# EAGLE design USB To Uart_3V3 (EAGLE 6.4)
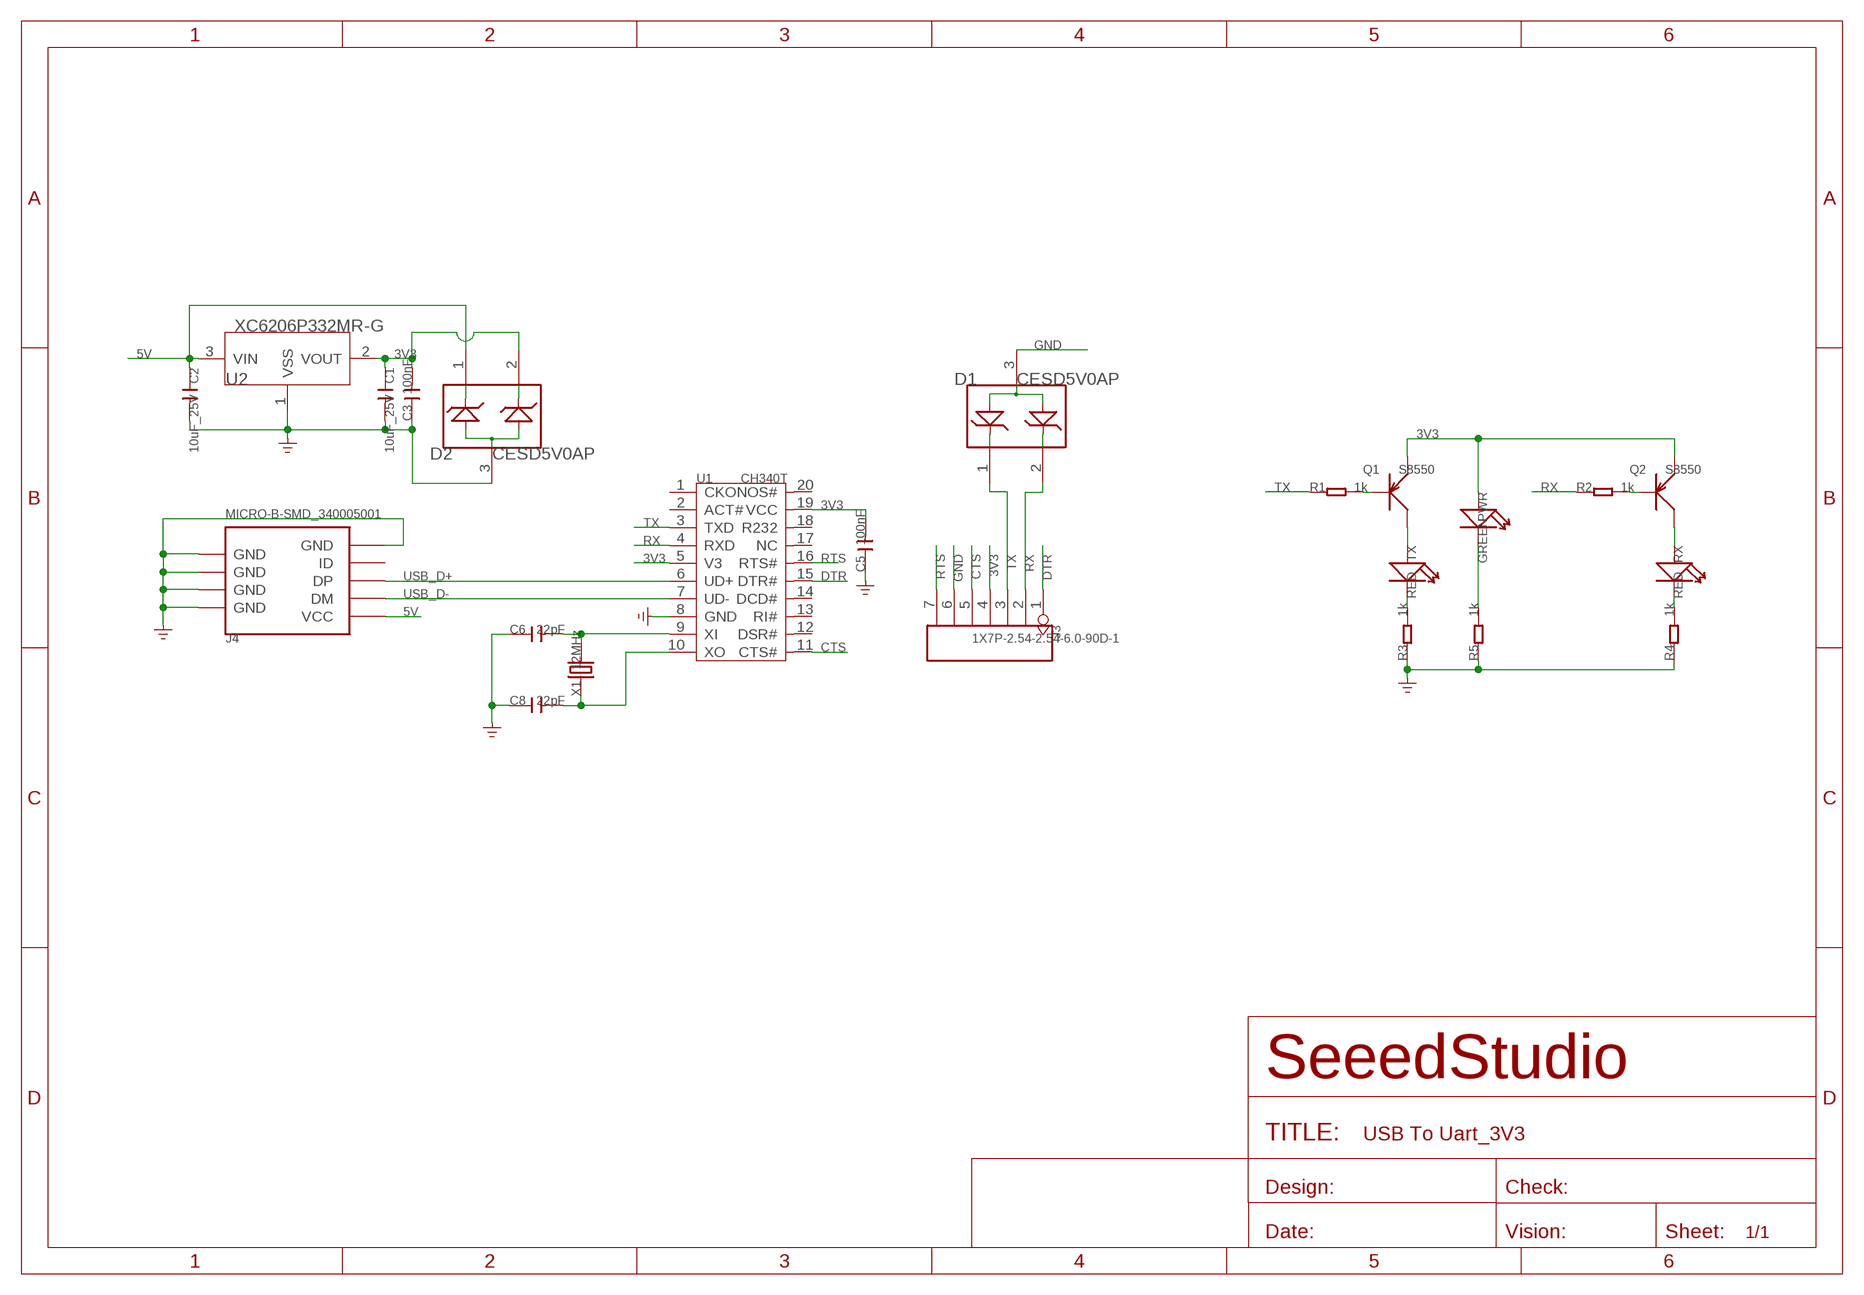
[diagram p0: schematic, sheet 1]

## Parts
C1  10uF_25V  C-0805  [C0805]
C2  10uF_25V  C-0805  [C0805]
C3  100nF  C-0402  [C0402]
C5  100nF  C-0402  [C0402]
C6  22pF  C-0402  [C0402]
C8  22pF  C-0402  [C0402]
D1  CESD5V0AP  D-ESD-3P  [SOT23]
D2  CESD5V0AP  D-ESD-3P  [SOT23]
J3  1X7P-2.54-2.54-6.0-90D-1  HEADER-7P  [7P-2.54-65/35MIL]
J4  MICRO-B-SMD_340005001  USB-MINIUSB-5P-MICRO  [MICRO-USB]
PWR  GREEN  LED'0603'  [LED-0603]
Q1  S8550  TRANSISTOR-PNP-SOT23  [SOT23]
Q2  S8550  TRANSISTOR-PNP-SOT23  [SOT23]
R1  1k  R-0402  [R0402]
R2  1k  R-0402  [R0402]
R3  1k  R-0402  [R0402]
R4  1k  R-0402  [R0402]
R5  1k  R-0402  [R0402]
RX  RED  LED'0603'  [LED-0603]
TX  RED  LED'0603'  [LED-0603]
U1  CH340T  [SSOP20]
U2  XC6206P332MR-G  XC6206MR  [SOT23]
X1  12MHz  CRYSTAL'HC49UP'  [HC49UP]

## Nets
3V3: C1.1 C3.2 C5.2 D2.2 J3.4 PWR.+ Q1.2(E) Q2.2(E) U1.5(V3) U1.19(VCC) U2.2(VOUT)
5V: C2.1 D2.1 J4.1(VCC) U2.3(VIN)
CTS: J3.5 U1.11(CTS#)
DTR: J3.1 U1.15(DTR#)
GND: C1.2 C2.2 C3.1 C5.1 C6.1 C8.1 D1.3 D2.3 J3.6 J4.5(GND) J4.S1(GND) J4.S2(GND) J4.S3(GND) J4.S4(GND) J4.S5(GND) J4.S6(GND) R3.1 R4.1 R5.1 U1.8(GND) U2.1(VSS)
N$1: Q1.3(C) TX.+
N$2: Q2.3(C) RX.+
N$4: C6.2 U1.9(XI) X1.2
N$5: C8.2 U1.10(XO) X1.1
N$6: R3.2 TX.-
N$7: Q1.1(B) R1.2
N$8: Q2.1(B) R2.2
N$10: R4.2 RX.-
N$12: PWR.- R5.2
RTS: J3.7 U1.16(RTS#)
RX: D1.2 J3.2 R2.1 U1.4(RXD)
TX: D1.1 J3.3 R1.1 U1.3(TXD)
USB_D+: J4.3(DP) U1.6(UD+)
USB_D-: J4.2(DM) U1.7(UD-)
Unconnected: J4.4(ID) U1.1(CKO) U1.2(ACT#) U1.12(DSR#) U1.13(RI#) U1.14(DCD#) U1.17(NC) U1.18(R232) U1.20(NOS#)

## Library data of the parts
C1-C3 C5 C6 C8 = Discrete:C*: Ceramic Capacitors
D1 D2 = Discrete:D-ESD-3P
J3 = Connector :HEADER-7P
J4 = Connector :USB-MINIUSB-5P
PWR RX TX = Discrete:LED*
Q1 Q2 = Discrete:TRANSISTOR-PNP*: PNP audion
R1-R5 = Discrete:R*
U1 = template:CH340T
U2 = IC:XC6206: LOW ESR Cap.Compatible Positive Voltage Regulators
X1 = Discrete:CRYSTAL*: CRYSTAL

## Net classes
0 default: width 0.152 mm, drill 0.305 mm, clearance 0.152 mm

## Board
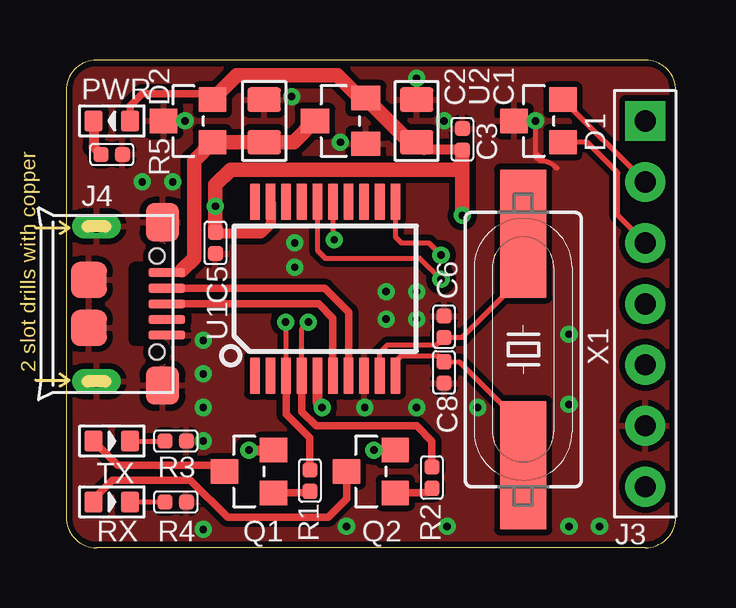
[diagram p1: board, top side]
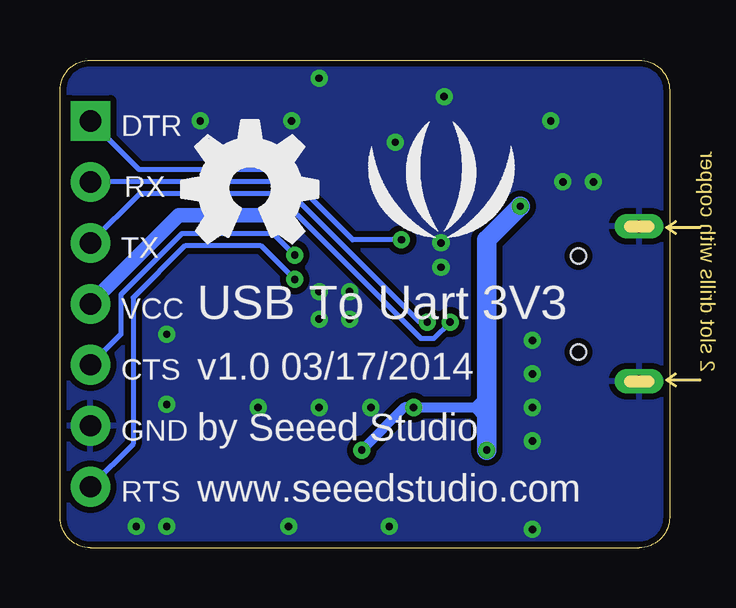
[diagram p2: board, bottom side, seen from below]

Size 25.4 x 20.32 mm. Coordinates in mm from the lower left corner, seen from the top.
Outline: 0,19.05 0,1.27 arc90 1.27,0 24.13,0 arc90 25.4,1.27 25.4,19.05 arc90 24.13,20.32 1.27,20.32 arc90 0,19.05
Copper layers (1*16): Top 0.035mm / dielectric 1.5mm / Bottom 0.035mm
Design rules "default *": minimum track width 8mil, minimum drill 12mil, track to track 8mil, track to pad 8mil, pad to pad 8mil, via to via 8mil, smd to smd 0mil, copper to edge 8mil, drill to drill 8mil, minimum pad ring 10mil, minimum via ring 8mil, stop-mask expansion 4mil, vias tented up to drill 25mil, thermal gap 10mil

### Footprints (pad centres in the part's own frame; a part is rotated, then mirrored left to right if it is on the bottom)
C0805 = smd 1.016 x 1.397: 1 -0.889,0; 2 0.889,0
C0402 = smd 0.635 x 0.635: 1 -0.445,0; 2 0.445,0
SOT23 = smd 1.016 x 1.143: 1 -0.889,-1.016; 2 0.889,-1.016; 3 0,1.016
7P-2.54-65/35MIL = drill 0.889 pad 1.651 square: 1 0,7.62 | drill 0.889 pad 1.651: 2 0,5.08; 3 0,2.54; 4 0,0; 5 0,-2.54; 6 0,-5.08; 7 0,-7.62
MICRO-USB = smd 0.381 x 1.524: 1 -1.3,-0.25; 2 -0.65,-0.25; 3 0,-0.25; 4 0.65,-0.25; 5 1.3,-0.25 | smd 1.6 x 1.397: S1 -3.4,-0.427; S6 3.4,-0.427 | drill 0.508 pad 1.016 long: S2 -3.226,-3.175; S5 3.226,-3.175 | smd 1.5 x 1.5: S3 -1,-3.5; S4 1,-3.5 | hole 0.635: -2,-0.65; 2,-0.65
LED-0603 = smd 0.762 x 0.889: + -0.762,0; - 0.762,0
R0402 = smd 0.635 x 0.635: 1 -0.445,0; 2 0.445,0
SSOP20 = smd 0.4 x 1.5: 1 -2.925,-3.625; 2 -2.275,-3.625; 3 -1.625,-3.625; 4 -0.975,-3.625; 5 -0.325,-3.625; 6 0.325,-3.625; 7 0.975,-3.625; 8 1.625,-3.625; 9 2.275,-3.625; 10 2.925,-3.625; 11 2.925,3.625; 12 2.275,3.625; 13 1.625,3.625; 14 0.975,3.625; 15 0.325,3.625; 16 -0.325,3.625; 17 -0.975,3.625; 18 -1.625,3.625; 19 -2.275,3.625; 20 -2.925,3.625
SOT23' = smd 1.016 x 1.2: 1 -0.95,-1.06; 2 0.95,-1.06; 3 0,1.06
HC49UP = smd 5.334 x 1.93: 1 -4.826,0; 2 4.826,0

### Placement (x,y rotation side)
C1  14.61,17.78 90 top
C2  8.26,17.78 90 top
C3  16.51,17.02 270 top
C5  6.22,12.7 90 top
C6  15.75,9.21 270 top
C8  15.75,7.3 90 top
D1  19.68,17.78 90 top
D2  5.08,17.78 90 top
J3  24.13,10.16 0 top
J4  4.45,10.16 270 top
PWR  1.91,17.78 180 top
Q1  7.62,3.17 90 top
Q2  12.7,3.17 90 top
R1  10.16,2.79 270 top
R2  15.24,2.92 270 top
R3  4.57,4.45 180 top
R4  4.57,1.91 180 top
R5  1.91,16.38 180 top
RX  1.91,1.91 0 top
TX  1.91,4.45 0 top
U1  10.79,10.79 0 top
U2  XC6206P332MR-G  [SOT23']  11.43,17.78 90 top
U$8  [LOGO_SILK]  9.53,14.61 0 bottom
U$9  [OSHW_FILLX200_NOTEXT]  20.32,12.7 0 bottom
X1  19.05,8.26 90 top

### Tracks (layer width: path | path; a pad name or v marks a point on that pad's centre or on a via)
3V3  (via drill 0.3, 0.3 pad 0.64)
  Top 0.305: D2.2 5.84,18.92 3.17,18.92 2.67,18.41 PWR.+
  Top 0.406: Q2.2 v12.83,4.06 | v7.62,4.06 Q1.2 | U1.5 10.47,6.04 v10.67,5.84 | U1.19 8.52,13.47 8.13,13.08 6.29,13.08 C5.2 | C3.2 14.92,16.57 C1.1
  Top 0.61: C1.1 14.33,16.89 U2.2 12.26,18.73 11.3,19.68 7.11,19.68 D2.2 | C3.2 16.51,16 | 16.51,16 16.26,15.75 6.86,15.75 6.22,15.11 v6.22,14.22 C5.2 | 16.51,16 v16.51,13.84
  Bottom 0.406: 8.13,5.84 v10.67,5.84 11.05,5.84 v12.83,4.06 | 8.13,5.84 7.62,6.35 | 8.13,5.84 7.75,5.46
  Bottom 0.61: v16.51,13.84 20.45,13.84 J3.4
  Bottom 0.813: v7.62,4.06 7.62,6.35 7.62,12.83 v6.22,14.22
5V
  Top 0.203: J4.1 4.73,11.46 4.83,11.56
  Top 0.61: 4.83,11.56 5.33,12.06 5.33,16.13 D2.1 C2.1 9.48,16.89 U2.3
CTS  (via drill 0.3)
  Top 0.203: U1.11 13.72,12.95 13.97,12.7 15.11,12.7 v15.62,12.19
  Bottom 0.203: v15.62,12.19 16.51,13.08 20.32,13.08 22.86,10.54 22.86,8.89 J3.5
DTR  (via drill 0.3)
  Top 0.203: U1.15 11.12,12.88 v11.18,12.83
  Bottom 0.203: v11.18,12.83 13.21,12.83 16.13,15.75 21.84,15.75 22.1,15.75 J3.1
GND  (via drill 0.3 pad 0.64)
  Top 0.203: v19.56,17.78 19.56,16.45 | 19.56,16.45 19.88,16.13 | 19.56,16.45 19.56,16.38 | 19.56,16.38 19.81,16.13 | 20.35,15.9 20.38,15.88 | 19.56,16.38 19.56,16.32 19.75,16.13 arc-45 20.4,15.86 20.45,15.81
  other vias: 5.71,4.45 5.71,0.76 15.88,0.89 11.68,0.89 22.23,0.89 9.53,12.7 5.71,7.24 5.71,5.84 4.45,15.24 9.4,18.8 14.61,19.56 15.75,17.78 3.17,15.24 20.95,0.89 11.43,16.89 13.34,10.67 14.61,10.67 9.53,11.68 13.34,9.53 14.61,9.53 4.95,17.78 12.45,5.84 14.61,5.84 5.71,8.64 17.14,5.84 20.95,5.97 20.95,8.89
  pour Top (isolate 0.254): 0,20.32 25.4,20.32 25.4,0 0,0
  pour Bottom (isolate 0.254): 0,20.32 25.4,20.32 25.4,0 0,0
N$1
  Top 0.305: TX.+ 2.16,3.43 6.35,3.43 Q1.3
N$2
  Top 0.305: RX.+ 1.14,2.03 1.93,2.82 5.18,2.82 6.73,1.27 10.92,1.27 11.68,2.03 Q2.3
N$4
  Top 0.203: U1.9 13.07,8.12 13.4,8.45 15.43,8.45 C6.2 16.51,8.76 18.92,11.18 18.92,12.95 X1.2
N$5
  Top 0.203: U1.10 13.72,7.75 13.97,8 15.49,8 C8.2 16.38,7.75 19.05,5.08 X1.1
N$6
  Top 0.203: TX.- R3.2
N$7
  Top 0.305: Q1.1 10.1,2.29 R1.2
N$8
  Top 0.305: Q2.1 15.05,2.29 R2.2
N$10
  Top 0.203: RX.- R4.2
N$12
  Top 0.406: PWR.- 1.14,16.7 R5.2
RTS  (via drill 0.3)
  Top 0.203: U1.16 10.47,12.39 10.79,12.06 14.73,12.06 v15.62,11.18
  Bottom 0.203: v15.62,11.18 17.02,12.57 20.19,12.57 22.35,10.41 22.35,4.32 J3.7
RX  (via drill 0.3)
  Top 0.203: 9.82,7.02 9.82,9.12 v10.1,9.4 | J3.2 D1.2
  Top 0.305: U1.4 9.82,7.02 9.82,5.67 10.41,5.08 14.61,5.08 15.24,4.45 R2.1
  Bottom 0.203: v10.1,9.4 10.41,9.4 16.26,15.24 J3.2
TX  (via drill 0.3)
  Top 0.203: D1.1 21.72,16.89 22.99,15.62 22.99,13.84 J3.3 | U1.3 9.17,9.37 v9.14,9.4
  Top 0.305: U1.3 9.17,5.56 10.16,4.57 R1.1
  Bottom 0.203: v9.14,9.4 9.82,8.72 10.38,8.72 16.39,14.74 22.09,14.74 J3.3
USB_D+
  Top 0.305: J4.3 10.53,10.16 11.12,9.57 U1.6
USB_D-
  Top 0.305: U1.7 11.77,9.81 10.77,10.81 J4.2

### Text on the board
bPlace: DTR | RX | TX | USB To Uart 3V3 | VCC | v1.0 03/17/2014 | CTS | by Seeed Studio | GND | www.seeedstudio.com | RTS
